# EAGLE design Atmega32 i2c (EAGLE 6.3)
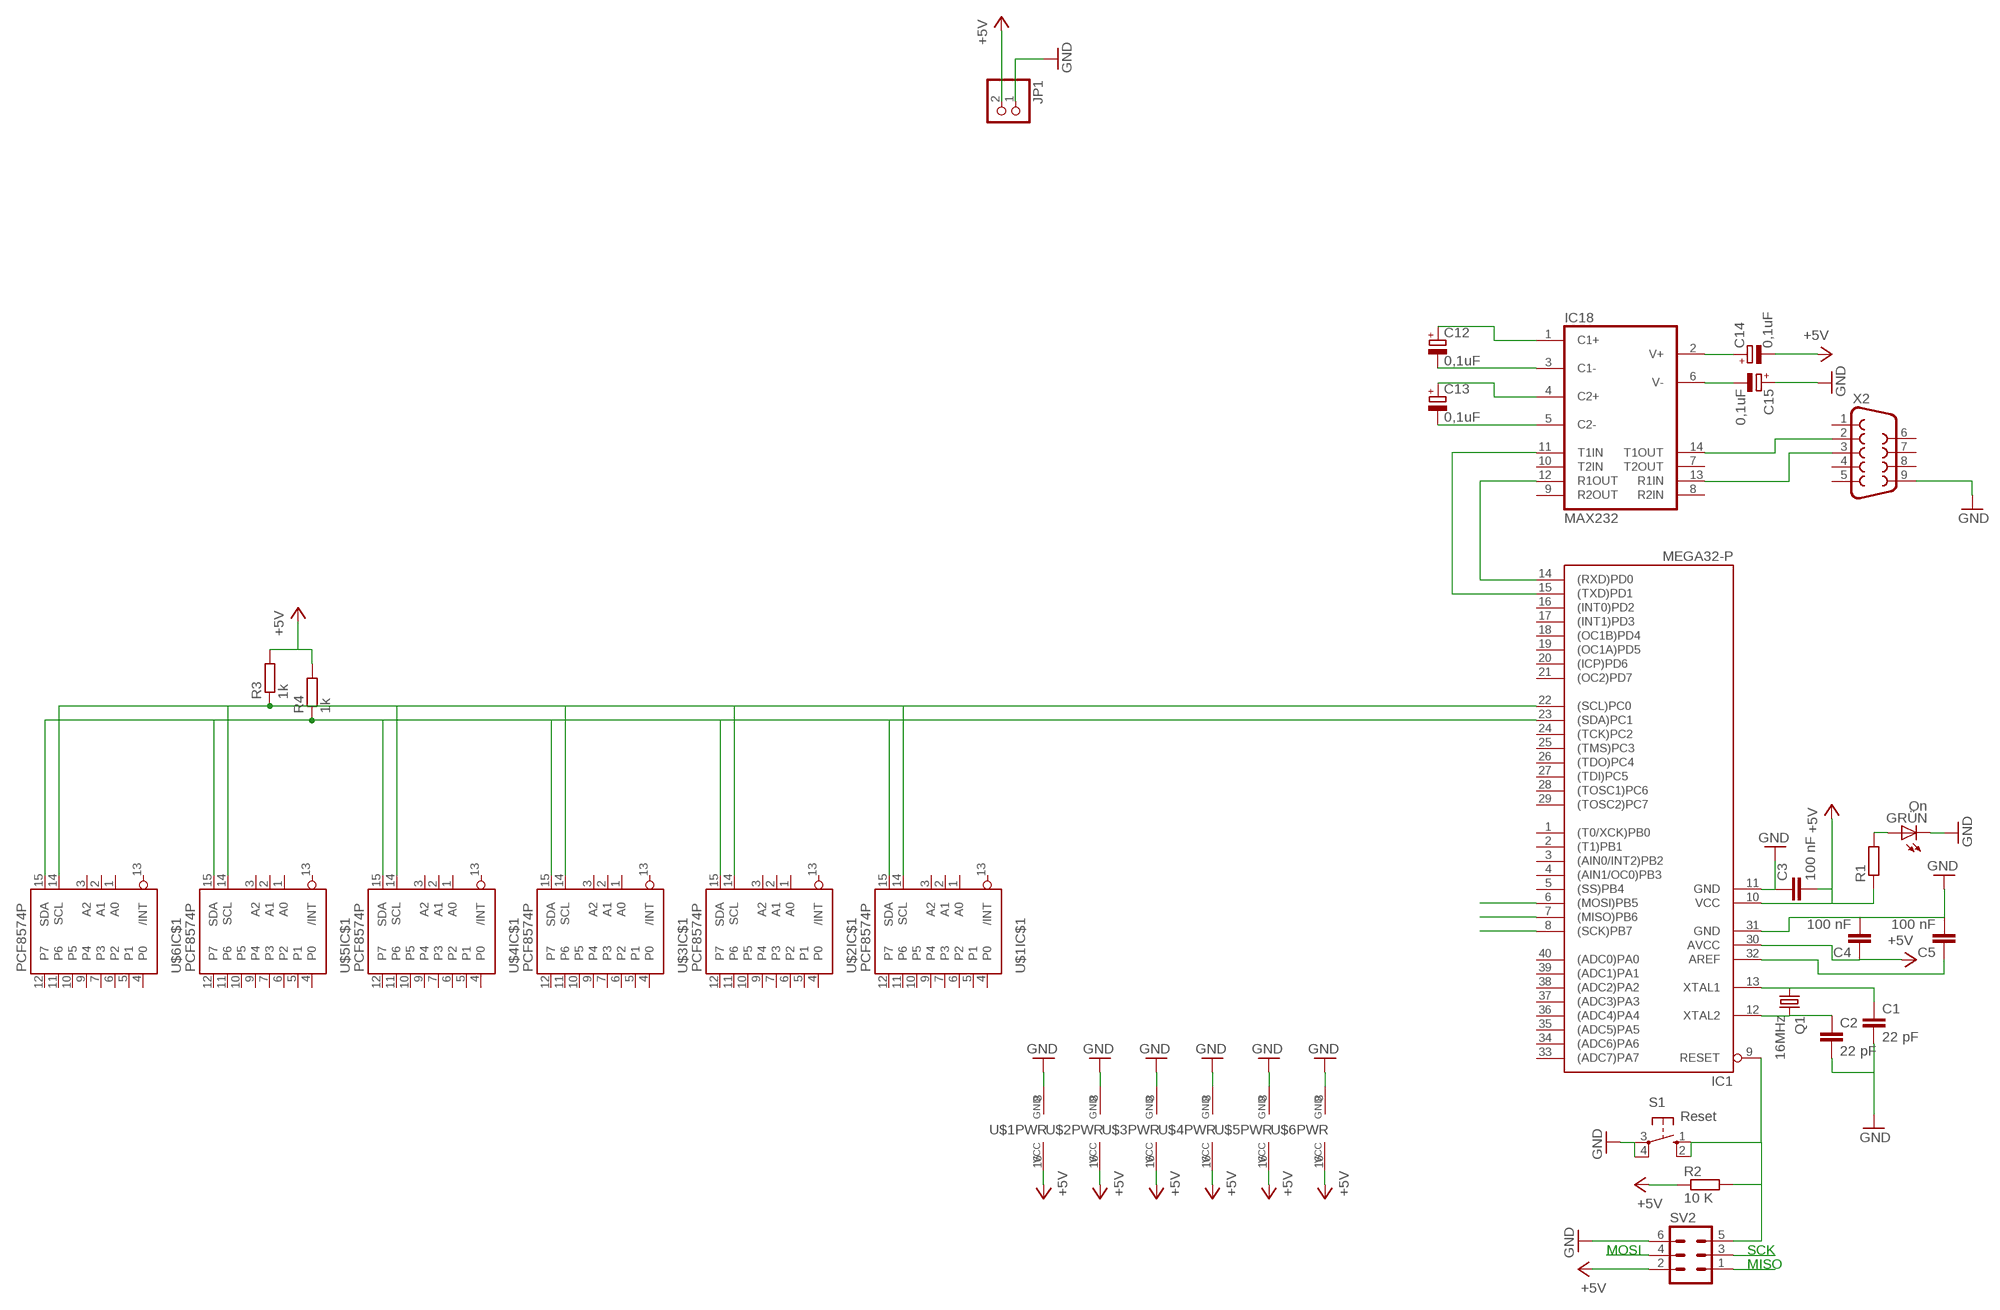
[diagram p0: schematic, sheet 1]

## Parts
C1  22 pF  C-EU025-024X044  [C025-024X044]
C2  22 pF  C-EU025-024X044  [C025-024X044]
C3  100 nF  C-EU025-024X044  [C025-024X044]
C4  100 nF  C-EU025-024X044  [C025-024X044]
C5  100 nF  C-EU025-024X044  [C025-024X044]
C12  0,1uF  CPOL-EUE2-5  [E2-5]
C13  0,1uF  CPOL-EUE2-5  [E2-5]
C14  0,1uF  CPOL-EUE2-5  [E2-5]
C15  0,1uF  CPOL-EUE2-5  [E2-5]
GRÜN  On  LED3MM  [LED3MM]
IC1  MEGA32-P  [DIL40]
IC18  MAX232  [DIL16]
JP1  PINHD-1X2  [1X02]
Q1  16MHz  CRYSTALHC49S  [HC49/S]
R1  R-EU_0204/7  [0204/7]
R2  10 K  R-EU_0207/2V  [0207/2V]
R3  1k  R-EU_0204/7  [0204/7]
R4  1k  R-EU_0204/7  [0204/7]
S1  Reset  10-XX  [B3F-10XX]
SV2  ML6  [ML6]
U$1  PCF8574P  [DIL16]
U$2  PCF8574P  [DIL16]
U$3  PCF8574P  [DIL16]
U$4  PCF8574P  [DIL16]
U$5  PCF8574P  [DIL16]
U$6  PCF8574P  [DIL16]
X2  F09HP  [F09HP]

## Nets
+5V: C3.2 C4.1 C14.- IC1.10(VCC) IC1.30(AVCC) JP1.2 R1.1 R2.1 R3.2 R4.2 SV2.2 U$1.16(PWR:VCC) U$2.16(PWR:VCC) U$3.16(PWR:VCC) U$4.16(PWR:VCC) U$5.16(PWR:VCC) U$6.16(PWR:VCC)
GND: C1.2 C2.2 C3.1 C4.2 C5.2 C15.+ GRÜN.K(C) IC1.11(GND) IC1.31(GND) JP1.1 S1.3(P) S1.4(P1) SV2.6 U$1.8(PWR:GND) U$2.8(PWR:GND) U$3.8(PWR:GND) U$4.8(PWR:GND) U$5.8(PWR:GND) U$6.8(PWR:GND) X2.9
MISO: IC1.7((MISO)PB6) SV2.1
N$1: C1.1 IC1.13(XTAL1) Q1.1
N$2: C2.1 IC1.12(XTAL2) Q1.2
N$3: GRÜN.A R1.2
N$4: C5.1 IC1.32(AREF)
N$5: IC1.23((SDA)PC1) R4.1 U$1.15(IC$1:SDA) U$2.15(IC$1:SDA) U$3.15(IC$1:SDA) U$4.15(IC$1:SDA) U$5.15(IC$1:SDA) U$6.15(IC$1:SDA)
N$6: IC1.22((SCL)PC0) R3.1 U$1.14(IC$1:SCL) U$2.14(IC$1:SCL) U$3.14(IC$1:SCL) U$4.14(IC$1:SCL) U$5.14(IC$1:SCL) U$6.14(IC$1:SCL)
N$7: IC1.9(RESET) R2.2 S1.1(S) S1.2(S1) SV2.5
N$17: IC1.15((TXD)PD1) IC18.11(T1IN)
N$18: IC1.14((RXD)PD0) IC18.12(R1OUT)
N$19: IC18.13(R1IN) X2.3
N$20: IC18.14(T1OUT) X2.2
N$21: C13.+ IC18.4(C2+)
N$22: C13.- IC18.5(C2-)
N$23: C12.- IC18.3(C1-)
N$24: C12.+ IC18.1(C1+)
N$25: C14.+ IC18.2(V+)
N$26: C15.- IC18.6(V-)
PB5: IC1.6((MOSI)PB5) SV2.4
SCK: IC1.8((SCK)PB7) SV2.3
Unconnected: IC1.1((T0/XCK)PB0) IC1.2((T1)PB1) IC1.3((AIN0/INT2)PB2) IC1.4((AIN1/OC0)PB3) IC1.5((SS)PB4) IC1.16((INT0)PD2) IC1.17((INT1)PD3) IC1.18((OC1B)PD4) IC1.19((OC1A)PD5) IC1.20((ICP)PD6) IC1.21((OC2)PD7) IC1.24((TCK)PC2) IC1.25((TMS)PC3) IC1.26((TDO)PC4) IC1.27((TDI)PC5) IC1.28((TOSC1)PC6) IC1.29((TOSC2)PC7) IC1.33((ADC7)PA7) IC1.34((ADC6)PA6) IC1.35((ADC5)PA5) IC1.36((ADC4)PA4) IC1.37((ADC3)PA3) IC1.38((ADC2)PA2) IC1.39((ADC1)PA1) IC1.40((ADC0)PA0) IC18.7(T2OUT) IC18.8(R2IN) IC18.9(R2OUT) IC18.10(T2IN) U$1.1(IC$1:A0) U$1.2(IC$1:A1) U$1.3(IC$1:A2) U$1.4(IC$1:P0) U$1.5(IC$1:P1) U$1.6(IC$1:P2) U$1.7(IC$1:P3) U$1.9(IC$1:P4) U$1.10(IC$1:P5) U$1.11(IC$1:P6) U$1.12(IC$1:P7) U$1.13(IC$1:/INT) U$2.1(IC$1:A0) U$2.2(IC$1:A1) U$2.3(IC$1:A2) U$2.4(IC$1:P0) U$2.5(IC$1:P1) U$2.6(IC$1:P2) U$2.7(IC$1:P3) U$2.9(IC$1:P4) U$2.10(IC$1:P5) U$2.11(IC$1:P6) U$2.12(IC$1:P7) U$2.13(IC$1:/INT) U$3.1(IC$1:A0) U$3.2(IC$1:A1) U$3.3(IC$1:A2) U$3.4(IC$1:P0) U$3.5(IC$1:P1) U$3.6(IC$1:P2) U$3.7(IC$1:P3) U$3.9(IC$1:P4) U$3.10(IC$1:P5) U$3.11(IC$1:P6) U$3.12(IC$1:P7) U$3.13(IC$1:/INT) U$4.1(IC$1:A0) U$4.2(IC$1:A1) U$4.3(IC$1:A2) U$4.4(IC$1:P0) U$4.5(IC$1:P1) U$4.6(IC$1:P2) U$4.7(IC$1:P3) U$4.9(IC$1:P4) U$4.10(IC$1:P5) U$4.11(IC$1:P6) U$4.12(IC$1:P7) U$4.13(IC$1:/INT) U$5.1(IC$1:A0) U$5.2(IC$1:A1) U$5.3(IC$1:A2) U$5.4(IC$1:P0) U$5.5(IC$1:P1) U$5.6(IC$1:P2) U$5.7(IC$1:P3) U$5.9(IC$1:P4) U$5.10(IC$1:P5) U$5.11(IC$1:P6) U$5.12(IC$1:P7) U$5.13(IC$1:/INT) U$6.1(IC$1:A0) U$6.2(IC$1:A1) U$6.3(IC$1:A2) U$6.4(IC$1:P0) U$6.5(IC$1:P1) U$6.6(IC$1:P2) U$6.7(IC$1:P3) U$6.9(IC$1:P4) U$6.10(IC$1:P5) U$6.11(IC$1:P6) U$6.12(IC$1:P7) U$6.13(IC$1:/INT) X2.1 X2.4 X2.5 X2.6 X2.7 X2.8

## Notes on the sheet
- MOSI | SCK
- MISO

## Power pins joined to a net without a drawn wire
GND: IC18.15(GND)
VCC: IC18.16(VCC)

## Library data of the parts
C1-C5 = resistor:C-EU: CAPACITOR, European symbol
C12-C15 = resistor:CPOL-EU: POLARIZED CAPACITOR, European symbol
GRÜN = led:LED: LED
IC1 = atmel:MEGA32-P: MICROCONTROLLER 32 Kbytes FLASH 2 Kbytes SRAM 1 Kbytes EEPROM USART 8-channel 10 bit ADC Source: www.atmel.com .. doc2503.pdf; MPN: ATMEGA32-16PU; OC_FARNELL: 1661729; OC_NEWARK: 51P1794
IC18 = maxim:MAX232: RS232 TRANSEIVER; MF: MAXIM; MPN: MAX232ACPE+; OC_FARNELL: 9723773; OC_NEWARK: 68K4544
JP1 = pinhead:PINHD-1X2: PIN HEADER
Q1 = crystal:CRYSTAL: CRYSTAL; OC_FARNELL: 1667008; OC_NEWARK: unknown
R1-R4 = resistor:R-EU_: RESISTOR, European symbol
S1 = switch-omron:10-XX: OMRON SWITCH; MPN: B3F-1000; OC_FARNELL: 176432; OC_NEWARK: 36M3542
SV2 = con-ml:ML6: HARTING; OC_FARNELL: unknown; OC_NEWARK: unknown
U$1-U$6 = i2c:PCF8574: Remote 8-Bit I/O Expander for I²C Bus
X2 = con-subd:F09: SUB-D; OC_FARNELL: unknown; OC_NEWARK: unknown

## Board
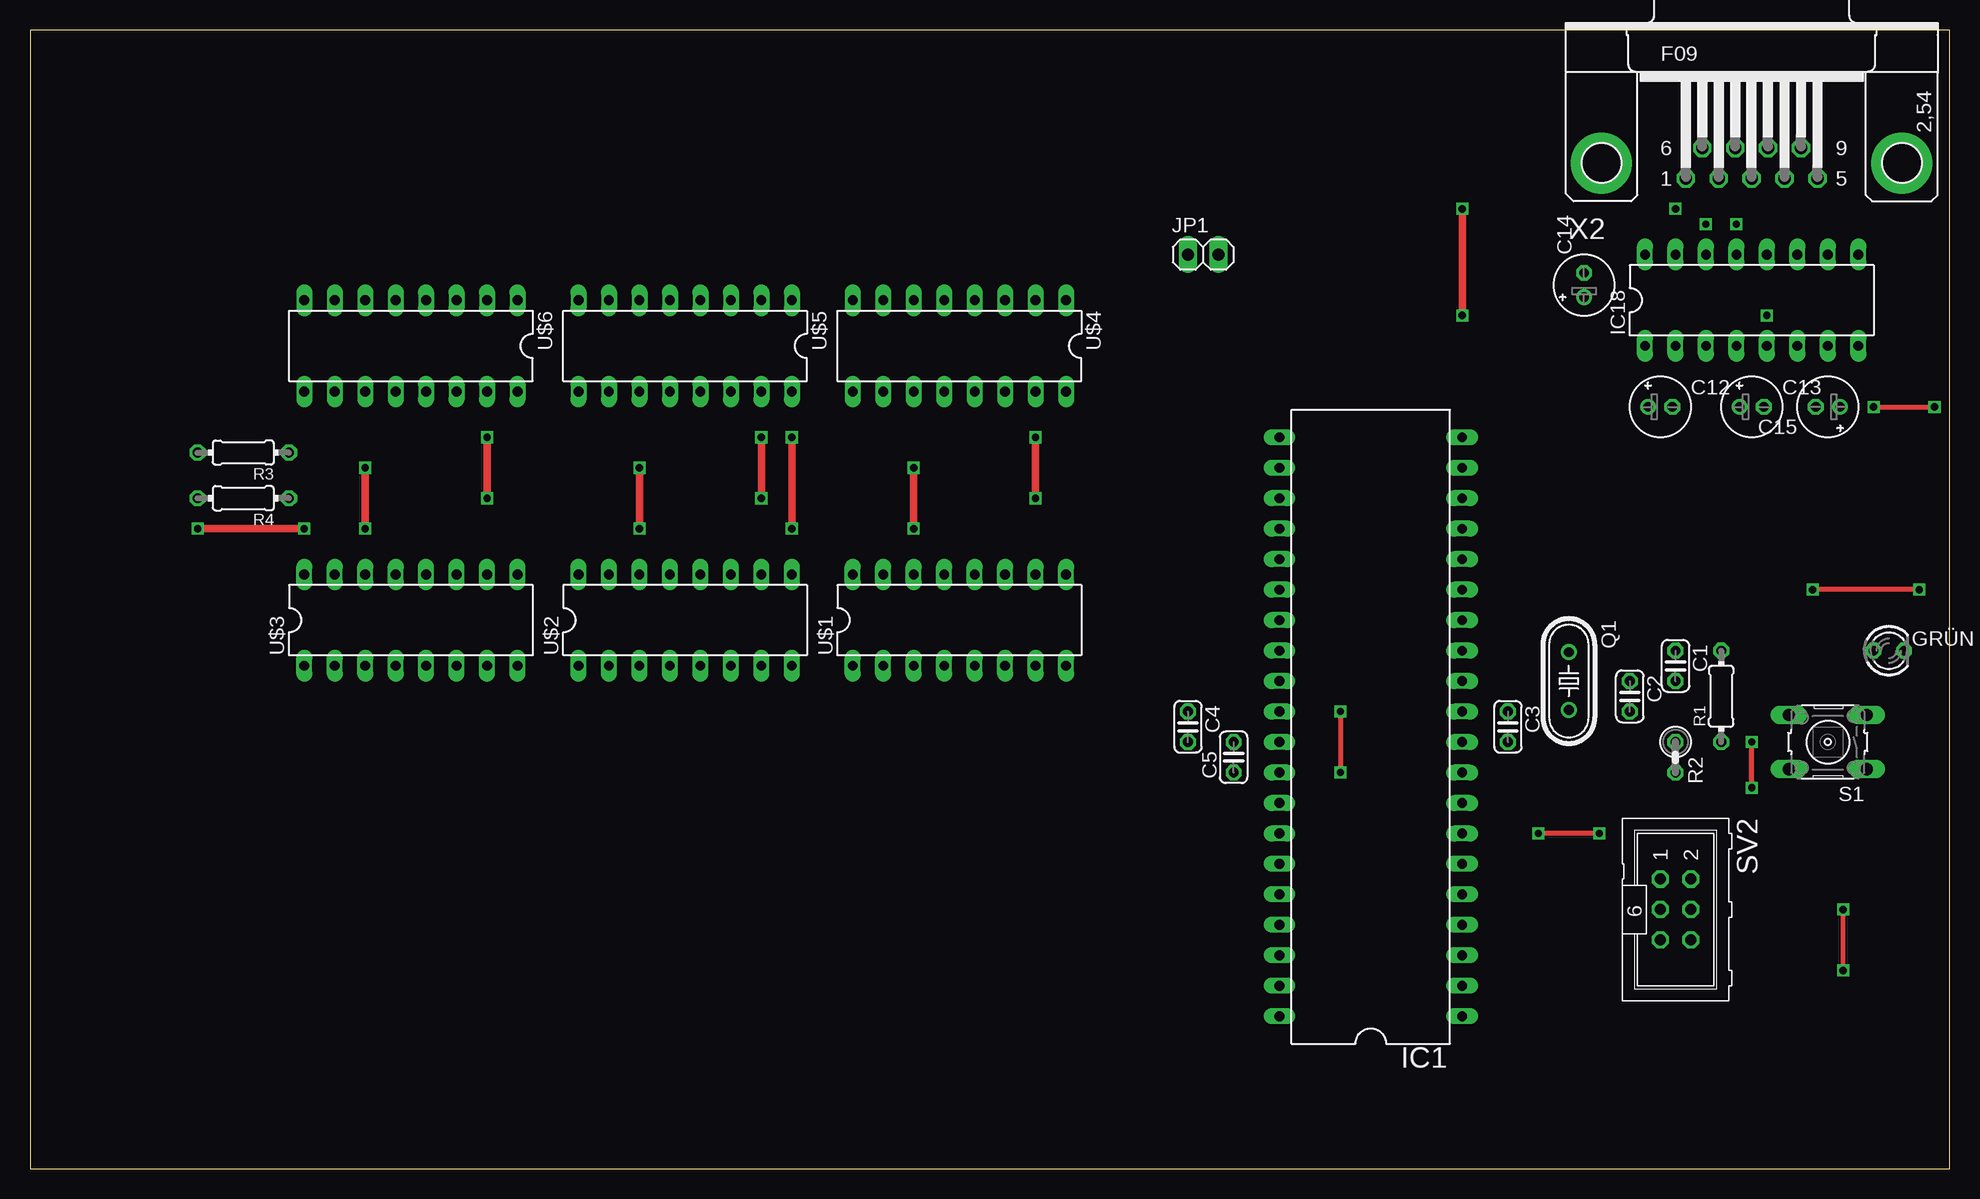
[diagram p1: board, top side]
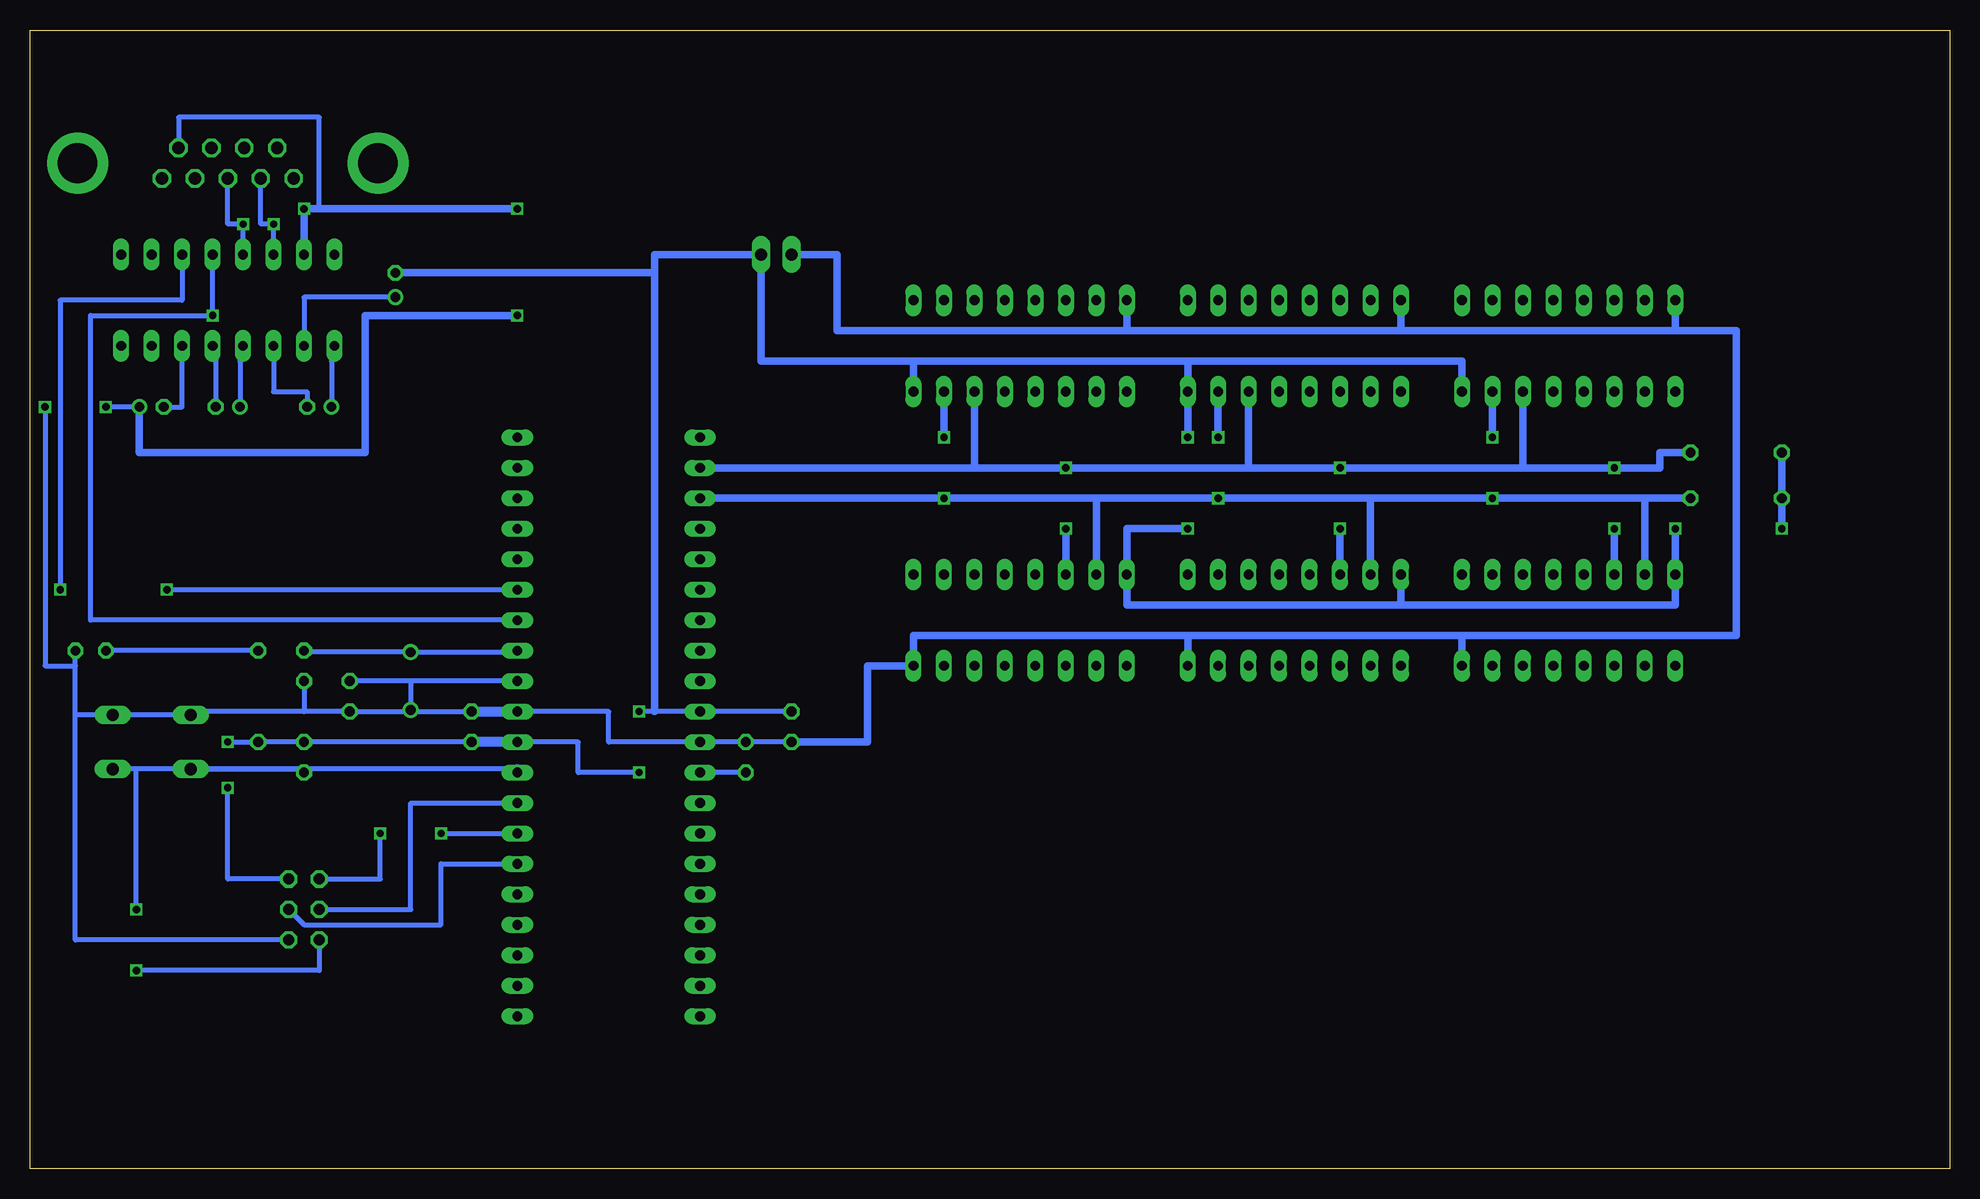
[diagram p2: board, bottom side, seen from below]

Size 160 x 94.92 mm. Coordinates in mm from the lower left corner, seen from the top.
Outline: 0,0 160,0 160,94.92 0,94.92 0,0
Copper layers (1*16): Top 0.035mm / dielectric 1.5mm / Bottom 0.035mm
Design rules "default": minimum track width 10mil, minimum drill 24mil, track to track 8mil, track to pad 8mil, pad to pad 8mil, via to via 8mil, smd to smd 8mil, copper to edge 40mil, drill to drill 8mil, minimum pad ring 10mil, minimum via ring 8mil, stop-mask expansion 4mil, vias tented up to drill 0mil, thermal gap 10mil

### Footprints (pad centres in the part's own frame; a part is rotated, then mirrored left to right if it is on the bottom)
C025-024X044 = drill 0.813 octagon: 1 -1.27,0; 2 1.27,0
E2-5 = drill 0.813 pad 1.27: + -1.016,0 | drill 0.813 pad 1.27 octagon: - 1.016,0
LED3MM = drill 0.813 octagon: A -1.27,0; K 1.27,0
DIL40 = drill 0.813 long: 1 -24.13,-7.62; 2 -21.59,-7.62; 3 -19.05,-7.62; 4 -16.51,-7.62; 5 -13.97,-7.62; 6 -11.43,-7.62; 7 -8.89,-7.62; 8 -6.35,-7.62; 9 -3.81,-7.62; 10 -1.27,-7.62; 11 1.27,-7.62; 12 3.81,-7.62; 13 6.35,-7.62; 14 8.89,-7.62; 15 11.43,-7.62; 16 13.97,-7.62; 17 16.51,-7.62; 18 19.05,-7.62; 19 21.59,-7.62; 20 24.13,-7.62; 21 24.13,7.62; 22 21.59,7.62; 23 19.05,7.62; 24 16.51,7.62; 25 13.97,7.62; 26 11.43,7.62; 27 8.89,7.62; 28 6.35,7.62; 29 3.81,7.62; 30 1.27,7.62; 31 -1.27,7.62; 32 -3.81,7.62; 33 -6.35,7.62; 34 -8.89,7.62; 35 -11.43,7.62; 36 -13.97,7.62; 37 -16.51,7.62; 38 -19.05,7.62; 39 -21.59,7.62; 40 -24.13,7.62
DIL16 = drill 0.813 long: 1 -8.89,-3.81; 2 -6.35,-3.81; 3 -3.81,-3.81; 4 -1.27,-3.81; 5 1.27,-3.81; 6 3.81,-3.81; 7 6.35,-3.81; 8 8.89,-3.81; 9 8.89,3.81; 10 6.35,3.81; 11 3.81,3.81; 12 1.27,3.81; 13 -1.27,3.81; 14 -3.81,3.81; 15 -6.35,3.81; 16 -8.89,3.81
1X02 = drill 1.016 long: 1 -1.27,0; 2 1.27,0
HC49/S = drill 0.813: 1 -2.413,0; 2 2.413,0
0204/7 = drill 0.813 octagon: 1 -3.81,0; 2 3.81,0
0207/2V = drill 0.813 octagon: 1 -1.27,0; 2 1.27,0
B3F-10XX = drill 1.016 long: 1 -3.251,2.261; 2 3.251,2.261; 3 -3.251,-2.261; 4 3.251,-2.261
ML6 = drill 0.914 octagon: 1 -2.54,-1.27; 2 -2.54,1.27; 3 0,-1.27; 4 0,1.27; 5 2.54,-1.27; 6 2.54,1.27
F09HP = drill 1.016 octagon: 1 -5.486,-1.27; 2 -2.743,-1.27; 3 0,-1.27; 4 2.743,-1.27; 5 5.486,-1.27; 6 -4.115,1.27; 7 -1.372,1.27; 8 1.372,1.27; 9 4.115,1.27 | drill 3.302 pad 5.08: G1 -12.522,0; G2 12.522,0

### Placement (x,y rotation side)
C1  137.16,41.91 270 top
C2  133.35,39.37 270 top
C3  123.19,36.83 270 top
C4  96.52,36.83 270 top
C5  100.33,34.29 90 top
C12  135.89,63.5 0 top
C13  143.51,63.5 0 top
C14  129.54,73.66 90 top
C15  149.86,63.5 180 top
GRÜN  154.94,43.18 0 top
IC1  111.76,36.83 90 top
IC18  143.51,72.39 0 top
JP1  97.79,76.2 0 top
Q1  128.27,40.64 270 top
R1  140.97,39.37 90 top
R2  137.16,34.29 270 top
R3  17.78,59.69 180 top
R4  17.78,55.88 180 top
S1  149.86,35.56 180 top
SV2  137.16,21.59 270 top
U$1  77.47,45.72 0 top
U$2  54.61,45.72 0 top
U$3  31.75,45.72 0 top
U$4  77.47,68.58 180 top
U$5  54.61,68.58 180 top
U$6  31.75,68.58 180 top
X2  143.51,83.82 0 top

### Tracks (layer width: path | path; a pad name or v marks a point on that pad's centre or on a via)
+5V  (via drill 0.6)
  Top 0.406: v143.51,31.75 v143.51,35.56 | v109.22,38.1 v109.22,33.02
  Top 0.61: v63.5,53.34 v63.5,60.96 | v13.97,53.34 v22.86,53.34
  Bottom 0.406: SV2.2 143.51,24.13 v143.51,31.75 | v143.51,35.56 R1.1 R2.1 C3.2 | C4.1 IC1.30 107.95,38.1 v109.22,38.1 | v109.22,33.02 114.3,33.02 114.3,35.56 IC1.10
  Bottom 0.61: 45.72,46.99 22.86,46.99 U$3.16 v22.86,53.34 | U$2.16 45.72,46.99 | 45.72,46.99 68.58,46.99 U$1.16 68.58,53.34 v63.5,53.34 | U$6.16 40.64,67.31 63.5,67.31 | 63.5,67.31 U$5.16 v63.5,60.96 | 63.5,67.31 86.36,67.31 | 86.36,67.31 U$4.16 | C14.- 107.95,74.68 | 107.95,74.68 107.95,38.1 | 86.36,67.31 99.06,67.31 JP1.2 107.95,76.2 107.95,74.68 | R4.2 R3.2 v13.97,53.34
  Bottom 0.813: IC1.10 C3.2
GND  (via drill 0.6)
  Top 0.406: v153.67,63.5 v158.75,63.5
  Top 0.61: v119.38,80.01 v119.38,71.12
  Bottom 0.406: 137.16,38.1 C2.2 C3.1 | C1.2 137.16,38.1 | 137.16,38.1 146.61,38.1 S1.4 S1.3 156.21,37.82 | 156.21,37.82 156.21,41.91 | 156.21,41.91 GRÜN.K | SV2.6 156.21,19.05 156.21,37.82 | v158.75,63.5 158.75,41.91 156.21,41.91 | C15.+ v153.67,63.5 | v137.16,80.01 135.89,80.01 135.89,87.63 147.62,87.63 X2.9 | C4.2 C5.2 IC1.31 111.76,35.56 111.76,38.1 IC1.11
  Bottom 0.61: U$6.8 22.86,69.85 | 22.86,69.85 45.72,69.85 | U$5.8 45.72,69.85 | 45.72,69.85 68.58,69.85 | U$4.8 68.58,71.12 68.58,69.85 | U$3.8 40.64,44.45 | 40.64,44.45 63.5,44.45 | U$2.8 63.5,44.45 | 63.5,44.45 86.36,44.45 U$1.8 90.17,41.91 90.17,35.56 C4.2 | 40.64,44.45 17.78,44.45 17.78,69.85 22.86,69.85 | IC18.15 v137.16,80.01 v119.38,80.01 | v119.38,71.12 132.08,71.12 132.08,59.69 150.88,59.69 C15.+ | JP1.1 92.71,76.2 92.71,69.85 68.58,69.85
  Bottom 0.813: C3.1 IC1.11
MISO  (via drill 0.6)
  Top 0.406: v130.81,27.94 v125.73,27.94
  Bottom 0.406: SV2.1 130.81,24.13 v130.81,27.94 | v125.73,27.94 IC1.7
N$1
  Bottom 0.406: C1.1 137.16,43.05 Q1.1 119.38,43.05 IC1.13
N$2
  Bottom 0.406: IC1.12 128.27,40.64 | 128.27,40.64 Q1.2 | 128.27,40.64 C2.1
N$3
  Bottom 0.406: R1.2 GRÜN.A
N$4
  Bottom 0.406: C5.1 IC1.32
N$5  (via drill 0.6)
  Top 0.61: v38.1,55.88 v38.1,60.96 | v60.96,55.88 v60.96,60.96 | v83.82,55.88 v83.82,60.96
  Bottom 0.61: IC1.23 v83.82,55.88 71.12,55.88 | 71.12,55.88 v60.96,55.88 48.26,55.88 | 25.4,55.88 v38.1,55.88 48.26,55.88 | U$2.15 48.26,55.88 | v38.1,60.96 U$6.15 | v60.96,60.96 U$5.15 | U$1.15 71.12,55.88 | v83.82,60.96 U$4.15 | U$3.15 25.4,55.88 | R4.1 25.4,55.88
N$6  (via drill 0.6)
  Top 0.61: v50.8,58.42 v50.8,53.34 | v27.94,58.42 v27.94,53.34 | v73.66,53.34 v73.66,58.42
  Bottom 0.61: U$6.14 35.56,58.42 | 35.56,58.42 v50.8,58.42 58.42,58.42 | 58.42,58.42 U$5.14 | 58.42,58.42 v73.66,58.42 81.28,58.42 | 81.28,58.42 U$4.14 | 81.28,58.42 IC1.22 | v50.8,53.34 U$2.14 | 35.56,58.42 v27.94,58.42 24.13,58.42 24.13,59.69 R3.1 | v27.94,53.34 U$3.14 | U$1.14 v73.66,53.34
N$7  (via drill 0.6)
  Top 0.406: v151.13,16.51 v151.13,21.59
  Bottom 0.406: 119.38,33.3 S1.2 | S1.2 151.13,33.3 | 151.13,33.3 S1.1 | SV2.5 135.89,16.51 v151.13,16.51 | v151.13,21.59 151.13,33.3 | S1.2 137.16,33.3 R2.2
  Bottom 0.813: 119.38,33.3 IC1.9
N$17  (via drill 0.6)
  Top 0.406: v157.48,48.26 v148.59,48.26
  Bottom 0.406: IC18.11 147.32,72.39 157.48,72.39 v157.48,48.26 | v148.59,48.26 IC1.15
N$18  (via drill 0.6)
  Bottom 0.406: IC1.14 154.94,45.72 154.94,71.12 v144.78,71.12 IC18.12
N$19  (via drill 0.6)
  Bottom 0.406: IC18.13 v142.24,78.74 143.51,78.74 X2.3
N$20  (via drill 0.6)
  Bottom 0.406: IC18.14 v139.7,78.74 140.77,78.74 X2.2
N$21
  Bottom 0.406: IC18.4 142.49,67.31 C13.+
N$22
  Bottom 0.406: IC18.5 144.53,67.31 C13.-
N$23
  Bottom 0.406: IC18.3 139.7,64.77 136.91,64.77 C12.-
N$24
  Bottom 0.406: IC18.1 134.87,67.31 C12.+
N$25
  Bottom 0.406: C14.+ 137.16,72.64 IC18.2
N$26
  Bottom 0.406: C15.- 147.32,63.5 IC18.6
PB5
  Bottom 0.406: SV2.4 137.16,20.32 125.73,20.32 125.73,25.4 IC1.6
SCK
  Bottom 0.406: SV2.3 128.27,21.59 128.27,30.48 IC1.8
